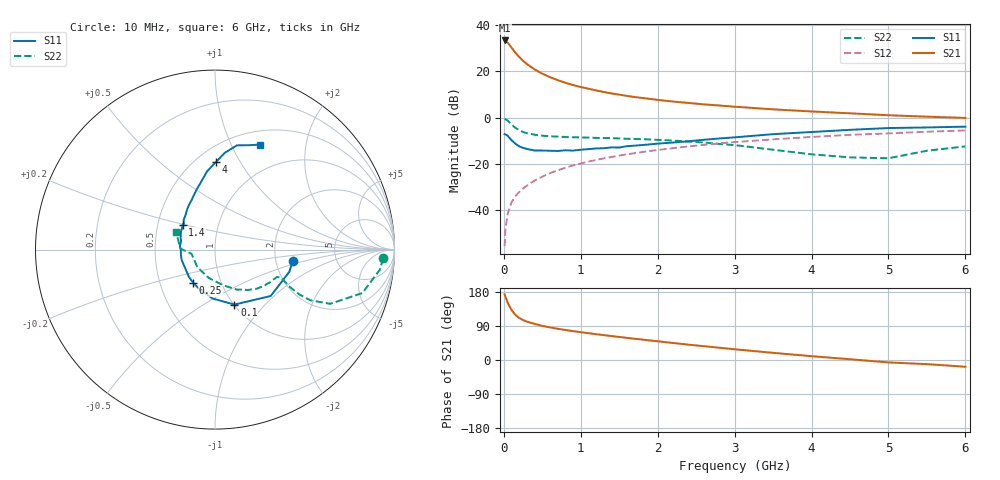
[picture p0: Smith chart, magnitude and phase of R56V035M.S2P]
! SIEMENS Small Signal Semiconductors
! BFR183
! Si NPN RF Bipolar Junction Transistor in SOT23
! VCE = 6 V  IC = 35 mA
! Common Emitter S-Parameters:  May  1996
# GHz  S  MA  R  50
!  f  S11  S21  S12  S22
! GHz  MAG  ANG  MAG  ANG  MAG  ANG  MAG  ANG
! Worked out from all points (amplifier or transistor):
!   36 points, 10 MHz to 6 GHz, reference 50 ohm
!   highest |S21| = 33.2 dB at 10 MHz (marker M1)
!   |S21| within 3 dB of that: start of sweep to 98.06 MHz
!   unconditionally stable (mu >= 1): 453.7 MHz to 2.408 GHz
!   at 250 MHz: K = 0.89, MSG = 27.5 dB, |S12| = -30.6 dB
!   at 1.4 GHz: K = 1.04, MAG = 12.4 dB, |S12| = -17.0 dB
!   at 6 GHz: K = 0.90, MSG = 2.7 dB, |S12| = -5.6 dB
!   S11 on the Smith chart (normalised r, x): 10 MHz: 2.48, -0.39; 100 MHz: 1.01, -0.69; 250 MHz: 0.74, -0.29; 1.4 GHz: 0.67, +0.19; 4 GHz: 0.62, +0.79; 6 GHz: 0.66, +1.29
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0.01  0.4368 -8.3  45.57 173.3  0.0017 94.4  0.938 -3.0
0.02  0.4325 -16.5  44.97 167.2  0.0038 78.8  0.9248 -7.0
0.05  0.4039 -39.8  40.89 151.3  0.0085 76.9  0.8566 -16.4
0.1  0.3249 -70.5  31.95 131.9  0.015 72.4  0.7094 -25.2
0.15  0.2729 -92.8  24.9 119.0  0.0203 70.8  0.6007 -28.0
0.2  0.2395 -109.9  20.05 111.1  0.0249 72.0  0.5341 -28.0
0.25  0.2218 -123.0  16.59 105.3  0.0296 71.9  0.488 -27.1
0.3  0.2107 -133.4  14.12 101.2  0.0341 73.0  0.4599 -26.3
0.4  0.1949 -150.0  10.88 95.3  0.0439 74.3  0.4261 -24.5
0.5  0.1946 -162.3  8.778 90.1  0.0533 74.7  0.4063 -23.5
0.6  0.1923 -170.8  7.39 86.1  0.0635 74.4  0.395 -23.2
0.8  0.197 173.9  5.606 79.2  0.0829 73.1  0.381 -23.7
0.9  0.1939 166.9  5.004 76.2  0.093 72.5  0.3759 -24.0
1.1  0.2088 156.0  4.158 70.9  0.1124 71.0  0.369 -26.3
1.4  0.227 142.9  3.298 63.1  0.1415 68.0  0.3593 -29.9
1.7  0.2479 132.6  2.762 56.1  0.1706 64.8  0.3447 -34.1
2.2  0.2893 119.7  2.205 44.9  0.2193 59.1  0.3193 -43.0
3.5  0.4381 95.8  1.499 18.9  0.3385 42.4  0.2025 -77.6
4  0.4874 89.5  1.35 10.1  0.3811 36.4  0.1613 -102.7
4.5  0.5431 84.1  1.232 2.0  0.4234 29.7  0.1387 -134.9
5.5  0.6108 72.2  1.042 -10.9  0.4937 18.1  0.1927 178.2
6  0.6357 66.9  0.98 -17.8  0.527 10.6  0.2392 155.4
